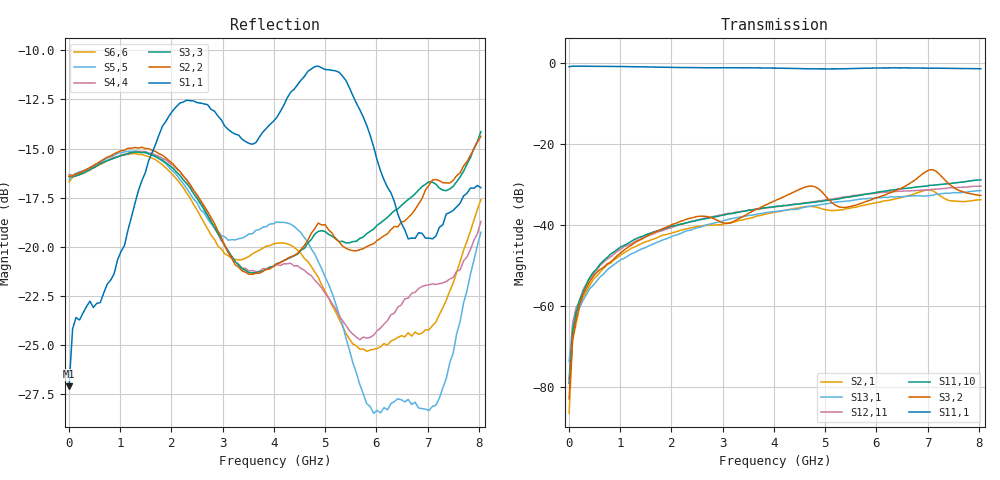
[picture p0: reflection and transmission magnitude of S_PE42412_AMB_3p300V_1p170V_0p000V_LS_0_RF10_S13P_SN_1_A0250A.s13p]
! Device ID: PE42412
! File Path: z:\PE42412\TE_GND_Post_Char_S-Param\All Parts\AMB\3p300\LS_0_RF10\PE42412_AMB_3p300V_1p170V_0p000V_LS_0_RF10_S13P_SN_1_A0250A.s13p
! Serial: 1
! Lot: A0250A
! Temp: AMB
! VDD: 3.300
! VSS: 0.000
! Control_Hi: 1.170
! Control_Lo: 0.000
! Logic State: LS_0_RF10
! Port 1:
! Port 2:
! Port 3:
! Port 4:
! Port 5:
! Port 6:
! Port 7:
! Port 8:
! Port 9:
! Port 10:
! Port 11:
! Port 12:
! Port 13:
! ThroughPath:1-11
! IDD: 0.0001070885
! ISS/IDD2: 4.76e-008
! IDMM3/IDD3: -2.307e-007
! Comment:
#  Hz  S  RI  R  50
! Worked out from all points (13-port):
!   120 points, 10 MHz to 8.037 GHz, reference 50 ohm
!   strongest paths, dB at 10 MHz, 2.034 GHz, 4.057 GHz, 6.08 GHz, 8.037 GHz:
!     S11,1: -0.9, -1.1, -1.3, -1.3, -1.4
!     S3,2: -83.0, -39.9, -33.9, -33.0, -32.8
!     S11,10: -79.2, -40.3, -35.4, -31.8, -28.9
!     S12,11: -78.1, -40.6, -35.5, -32.1, -30.5
!     S13,1: -73.8, -42.8, -36.7, -33.3, -31.6
!     S2,1: -86.6, -42.0, -36.9, -34.4, -33.8
!   lowest |S11| = -27.1 dB at 10 MHz (marker M1), VSWR 1.09, Z = 53.5 - j2.98 ohm
!   |S11| at or under -10 dB: start of sweep to end of sweep
